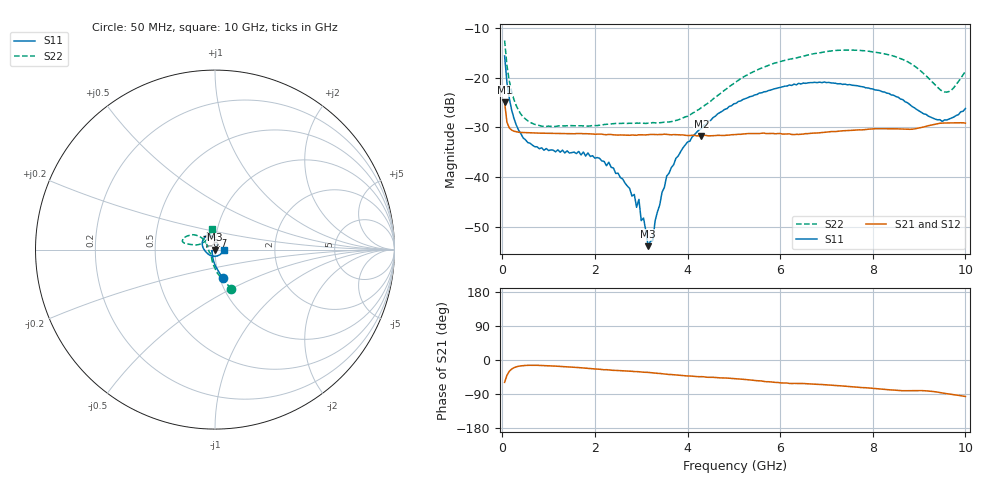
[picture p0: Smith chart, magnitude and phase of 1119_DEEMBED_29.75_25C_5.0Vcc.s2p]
!Hittite Microwave Corp.
!Digital Attenuator/PhaseShifter Rev 1.4.0
!Filename: C:\DATA\DATA\1119_DEEMBED_29.75_25C_5.0Vcc.s2p
!VNA ID: Agilent Technologies,N5224A,MY51441122,A.10.45.03
!Device type:
!2 Port Calibration.
!Temp(C): 25
!Lot Number:
!Serial Number:
!Operator:
!Misc:
!Attenuator:  29.750
# GHZ S DB R 50.0
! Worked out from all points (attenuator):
!   200 points, 50 MHz to 10 GHz, reference 50 ohm
!   highest |S21| = -24.92 dB at 50 MHz (marker M1); lowest = -31.7 dB at 4.3 GHz (marker M2)
!   lowest |S11| = -53.8 dB at 3.15 GHz (marker M3), VSWR 1.00, Z = 49.8 - j0.0406 ohm
!   |S11| at or under -10 dB: start of sweep to end of sweep
!   |S22| runs from -29.8 to -12.6 dB; largest |S21 - S12| = 0.0001
!   S11 on the Smith chart (normalised r, x): 50 MHz: 1.03, -0.34; 6.7 GHz: 0.90, +0.14; 10 GHz: 1.10, -0.00
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0.05  -15.65 -75.1  -24.92 -59.0  -24.92 -59.1  -12.56 -67.5
0.1  -20.95 -89.1  -28.93 -40.5  -28.95 -40.6  -17.51 -84.0
0.2  -26.41 -104.4  -30.51 -24.0  -30.52 -24.0  -22.78 -100.6
0.45  -32.08 -127.8  -31.01 -14.9  -31.02 -14.8  -27.87 -121.4
1.75  -34.92 -158.6  -31.25 -21.1  -31.24 -21.2  -29.67 -140.9
2.3  -36.95 -161.4  -31.38 -26.1  -31.39 -26.1  -29.30 -149.4
2.85  -43.41 -150.2  -31.52 -30.6  -31.52 -30.7  -29.17 -158.0
2.9  -45.99 -145.9  -31.56 -30.6  -31.56 -30.6  -29.12 -159.2
2.95  -44.41 -147.5  -31.46 -31.0  -31.47 -31.1  -29.14 -160.2
3  -48.65 -152.2  -31.46 -31.7  -31.46 -31.8  -29.12 -161.8
3.05  -48.14 -155.2  -31.48 -32.2  -31.50 -32.2  -29.16 -163.0
3.15  -53.78 -168.5  -31.44 -32.6  -31.45 -32.7  -29.13 -166.2
3.25  -52.60 105.7  -31.39 -34.2  -31.39 -34.2  -29.02 -169.0
3.4  -45.50 91.5  -31.40 -35.5  -31.41 -35.5  -29.05 -173.8
3.55  -39.72 78.3  -31.39 -37.8  -31.37 -37.9  -28.93 -179.2
3.75  -36.16 74.9  -31.43 -39.7  -31.43 -39.7  -28.58 172.9
4.3  -30.20 72.3  -31.69 -43.9  -31.69 -44.0  -25.99 150.3
5.05  -25.15 83.9  -31.41 -49.4  -31.42 -49.5  -20.83 138.6
6.7  -21.01 120.8  -31.13 -63.5  -31.14 -63.5  -15.26 153.8
8.35  -23.18 168.2  -30.27 -78.5  -30.27 -78.6  -15.44 168.1
9.55  -28.47 -70.5  -29.10 -88.0  -29.11 -88.0  -22.89 138.1
10  -26.19 -0.9  -29.12 -96.2  -29.11 -96.3  -18.75 98.2
